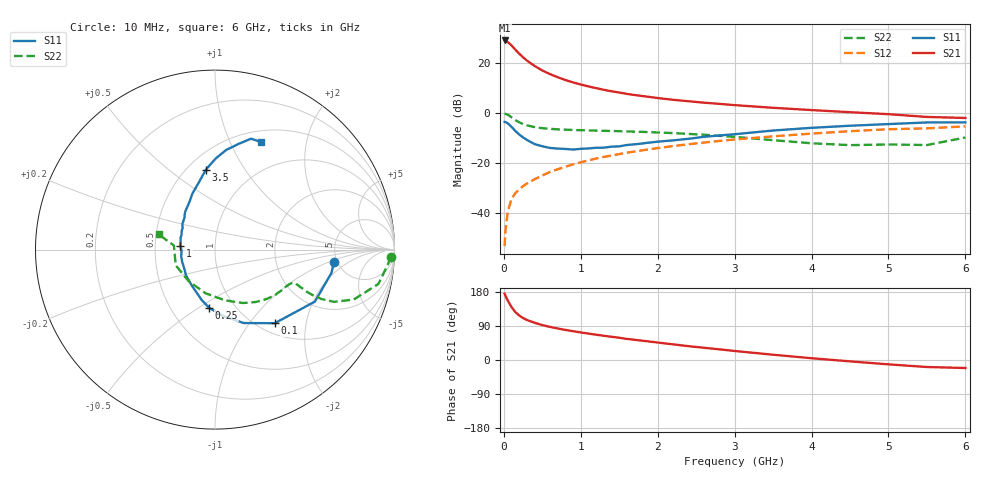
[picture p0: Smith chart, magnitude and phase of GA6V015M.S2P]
! Infineon Technologies  Discrete & RF Semiconductors
! BF775
! Si NPN RF Bipolar Junction Transistor in SOT23
! VCE = 6 V  IC = 15 mA
! Common Emitter S-Parameters:  May  1996
# GHz  S  MA  R  50
!  f  S11  S21  S12  S22
! GHz  MAG  ANG  MAG  ANG  MAG  ANG  MAG  ANG
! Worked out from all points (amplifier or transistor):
!   36 points, 10 MHz to 6 GHz, reference 50 ohm
!   highest |S21| = 29.0 dB at 10 MHz (marker M1)
!   |S21| within 3 dB of that: start of sweep to 129.6 MHz
!   unconditionally stable (mu >= 1): 487.9 MHz to 2.904 GHz
!   at 250 MHz: K = 0.77, MSG = 25.7 dB, |S12| = -29.2 dB
!   at 1.4 GHz: K = 1.10, MAG = 10.9 dB, |S12| = -17.0 dB
!   at 6 GHz: K = 0.91, MSG = 1.7 dB, |S12| = -5.3 dB
!   S11 on the Smith chart (normalised r, x): 10 MHz: 4.71, -1.14; 100 MHz: 1.18, -1.34; 250 MHz: 0.76, -0.55; 1 GHz: 0.68, +0.03; 3.5 GHz: 0.61, +0.68; 6 GHz: 0.63, +1.32
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0.01  0.6668 -5.8  28.17 174.8  0.0022 90.9  0.9806 -2.4
0.02  0.6615 -11.4  27.75 170.1  0.0043 80.3  0.9664 -5.0
0.05  0.6275 -27.5  26.28 157.4  0.0106 77.9  0.9299 -11.9
0.1  0.5284 -50.9  22.41 139.7  0.0194 69.9  0.8214 -19.8
0.15  0.4395 -68.6  18.4 126.4  0.0252 65.9  0.7244 -23.7
0.2  0.3736 -82.8  15.33 117.5  0.0299 65.0  0.6537 -24.9
0.25  0.3262 -95.7  12.97 110.6  0.0348 64.9  0.602 -25.0
0.3  0.2908 -104.7  11.18 105.6  0.0391 65.9  0.5673 -24.7
0.4  0.2401 -121.9  8.718 98.3  0.0478 66.7  0.525 -23.8
0.5  0.2175 -137.4  7.085 92.1  0.0567 67.9  0.4991 -23.1
0.6  0.2012 -148.5  5.994 87.4  0.0667 68.5  0.4839 -23.0
0.7  0.1954 -159.3  5.197 83.1  0.0755 68.7  0.4737 -23.2
0.8  0.1922 -168.2  4.568 79.4  0.0847 68.5  0.4658 -23.7
1  0.1934 173.7  3.717 72.7  0.1039 67.9  0.4552 -25.3
1.1  0.1966 167.2  3.407 69.7  0.1135 67.7  0.4508 -26.5
1.3  0.2037 156.1  2.914 64.0  0.133 66.2  0.4418 -28.8
1.6  0.2305 142.1  2.413 55.7  0.1616 63.9  0.4293 -33.1
2.2  0.285 122.5  1.841 41.3  0.2193 58.3  0.3983 -43.7
3.5  0.4483 96.5  1.274 13.9  0.343 43.4  0.2876 -79.1
4.5  0.5586 83.6  1.041 -3.6  0.4349 30.7  0.2289 -129.6
5.5  0.6497 72.0  0.837 -18.5  0.4952 15.6  0.23 174.3
6  0.6518 66.7  0.798 -21.1  0.5427 11.5  0.3248 164.9
